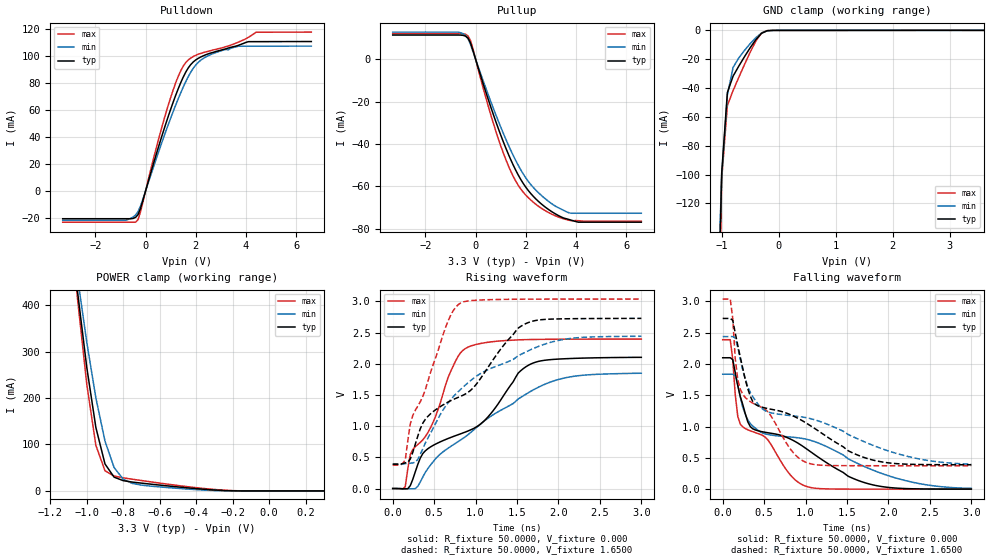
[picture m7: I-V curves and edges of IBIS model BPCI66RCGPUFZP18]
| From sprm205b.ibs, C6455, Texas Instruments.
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|   Model BPCI66RCGPUFZP18
[Model]   BPCI66RCGPUFZP18
Model_type   I/O
Polarity   Non-Inverting
Enable   Active-Low
Vinl =   0.8000V
Vinh =   2.0000V
Vmeas =   1.5000V
Cref =  10.0000pF
Rref =  50.0000
Vref =   1.5000V
C_comp   1.2405pF   1.1811pF   1.2768pF
[Temperature Range]   25.0000   0.1250k   -40.0000
[Pullup Reference]   3.3000V   3.0000V   3.6000V
[Pulldown Reference]   0.000V   0.000V   0.000V
[POWER Clamp Reference]   3.3000V   3.0000V   3.6000V
[GND Clamp Reference]   0.000V   0.000V   0.000V
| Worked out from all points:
|   slope of the pulldown table from 0 to 0.495 V, typ, clamps not added: 15.7 ohm
|   slope of the pullup table from 0 to 0.495 V, typ, clamps not added: 26.6 ohm
|   GND clamp passes 1 mA (typ) near -0.24 V on its own axis
|   POWER clamp passes 1 mA (typ) near -0.26 V on its own axis
|   rising waveform, R_fixture 50.0000, V_fixture 0.000: 20-80 % time 1.12ns typ, 1.11ns min, 510ps max; typ from 0 V to 2.1 V
|   rising waveform, R_fixture 50.0000, V_fixture 1.6500: 20-80 % time 1.01ns typ, 966ps min, 420ps max; typ from 0.391 V to 2.73 V
|   falling waveform, R_fixture 50.0000, V_fixture 0.000: 20-80 % time 1.08ns typ, 1.47ns min, 557ps max; typ from 2.1 V to 0.001 V
|   falling waveform, R_fixture 50.0000, V_fixture 1.6500: 20-80 % time 1.05ns typ, 1.4ns min, 563ps max; typ from 2.73 V to 0.39 V
[Pulldown]
| voltage   I(typ)   I(min)   I(max)
-3.3V     -20.59mA   -21.72mA   -23.16mA
-600mV    -20.59mA   -20.43mA   NA
-300mV    -17.52mA   -15.3mA    -21.29mA
500mV     31.76mA    27.95mA    37.14mA
1V        60.62mA    54.04mA    69.37mA
1.4V      80.3mA     72.79mA    89.13mA
1.8V      93.75mA    88.11mA    98.59mA
2.1V      98.38mA    95.39mA    101.4mA
2.4V      101mA      99.37mA    103.1mA
3.6V      107.4mA    106.9mA    109.6mA
4.1V      110.7mA    NA         114mA
6.6V      110.8mA    107.4mA    117.8mA
[Pullup]
| voltage   I(typ)   I(min)   I(max)
-3.3V     11.35mA    12.74mA    12mA
-700mV    11.35mA    12.74mA    NA
-300mV    9.868mA    9.624mA    10.87mA
-200mV    7.599mA    6.843mA    8.667mA
-100mV    3.916mA    3.444mA    4.629mA
700mV     -25.84mA   -22.95mA   -29.93mA
1.2V      -41.79mA   -37.61mA   -47.19mA
1.7V      -54.62mA   -50.05mA   -59.47mA
2.4V      -65.88mA   -61.73mA   -68.39mA
3.1V      -72.36mA   -68.68mA   -73.41mA
3.8V      -75.86mA   -72.62mA   -76.12mA
6.6V      -76.83mA   -72.62mA   -76.42mA
[GND_clamp]
| voltage   I(typ)   I(min)   I(max)
-3.3V     -13.5A     -11.41A    -15.22A
-1.1V     -266.1mA   -222mA     -325.5mA
-1V       -99.27mA   -101.4mA   -103.3mA
-900mV    -43.16mA   -44.9mA    -52.16mA
-800mV    -31.79mA   -25.73mA   -41.79mA
-700mV    -24.84mA   -19.16mA   -32.66mA
-500mV    -12.09mA   -9.237mA   -15.2mA
-400mV    -6.432mA   -5.07mA    -7.425mA
-300mV    -2.069mA   -1.879mA   -1.783mA
-200mV    -245.7uA   -339.8uA   -152.1uA
-100mV    -26.1uA    -33.32uA   -56.47uA
3.6V      0A         0A         0A
[POWER_clamp]
| voltage   I(typ)   I(min)   I(max)
-3.3V     9.99A      8.517A     11.3A
-1.1V     605.2mA    607.4mA    616.4mA
-1.05V    427.4mA    458.5mA    411.6mA
-1V       266.6mA    320.7mA    230.3mA
-950mV    136.8mA    200.5mA    98.27mA
-900mV    58.15mA    107.4mA    43.44mA
-850mV    29.68mA    50.44mA    32.02mA
-800mV    22.13mA    25.23mA    28.2mA
-750mV    19.05mA    16.21mA    25.23mA
-700mV    16.77mA    12.55mA    22.38mA
-250mV    883.2uA    290.5uA    1.647mA
300mV     0A         0A         0A
[Ramp]
| variable   typ   min   max
dV/dt_r   1.2618/1.1131n   1.1089/1.1325n   1.4371/0.5049n
dV/dt_f   1.5011/1.0265n   1.3191/1.3258n   1.6950/0.5906n
R_load = 50.0000
[Rising Waveform]
R_fixture = 50.0000
V_fixture = 0.000
V_fixture_min = 0.000
V_fixture_max = 0.000
| time   V(typ)   V(min)   V(max)
0s        202.5uV    70.43uV    561.2uV
151.5ps   -4.861mV   -2.417mV   31.43mV
212.1ps   46.11mV    -4.348mV   544.7mV
393.9ps   605.3mV    259.5mV    832.7mV
697ps     817.1mV    672.6mV    1.87V
878.8ps   906.9mV    832.9mV    2.245V
1.121ns   1.108V     1.1V       2.339V
1.515ns   1.852V     1.436V     2.384V
1.697ns   2.013V     1.582V     2.389V
3ns       2.103V     1.848V     2.396V
[Rising Waveform]
R_fixture = 50.0000
V_fixture = 1.6500
V_fixture_min = 1.5000
V_fixture_max = 1.8000
| time   V(typ)   V(min)   V(max)
0s        390.9mV    391.9mV    376.2mV
151.5ps   412mV      399.7mV    459.7mV
212.1ps   473.2mV    405.2mV    1.037V
242.4ps   581.7mV    411.3mV    1.171V
393.9ps   1.11V      729.1mV    1.586V
666.7ps   1.386V     1.371V     2.681V
818.2ps   1.478V     1.588V     2.973V
1.606ns   2.644V     2.189V     3.036V
2.121ns   2.722V     2.402V     3.037V
3ns       2.728V     2.441V     3.037V
[Falling Waveform]
R_fixture = 50.0000
V_fixture = 0.000
V_fixture_min = 0.000
V_fixture_max = 0.000
| time   V(typ)   V(min)   V(max)
0s        2.098V     1.836V     2.386V
90.91ps   2.098V     1.836V     2.386V
121.2ps   2.068V     1.836V     2.071V
181.8ps   1.657V     1.664V     1.163V
212.1ps   1.478V     1.472V     1.037V
363.6ps   963.6mV    1.007V     916.9mV
545.5ps   900.8mV    873mV      785mV
939.4ps   708.8mV    814.6mV    86.02mV
1.758ns   86.95mV    334.3mV    685.9uV
3ns       978.9uV    13.09mV    324uV
[Falling Waveform]
R_fixture = 50.0000
V_fixture = 1.6500
V_fixture_min = 1.5000
V_fixture_max = 1.8000
| time   V(typ)   V(min)   V(max)
0s        2.726V     2.436V     3.035V
90.91ps   2.726V     2.437V     3.034V
121.2ps   2.695V     2.437V     2.724V
151.5ps   2.493V     2.411V     2.081V
212.1ps   2.108V     2.077V     1.594V
363.6ps   1.395V     1.477V     1.373V
545.5ps   1.286V     1.233V     1.234V
939.4ps   1.109V     1.156V     476mV
1.788ns   473.4mV    713.3mV    374.5mV
3ns       389.9mV    401.3mV    374.1mV
